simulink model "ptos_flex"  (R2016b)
settings: Solver=ode4  StartTime=0.0  StopTime=trun  FixedStep=step_sz  RelTol=1e-7  EnableMultiTasking=on
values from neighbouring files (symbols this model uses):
  A = [0 1;-(w)^2 0;]    [figure_4.m]    (also in figure_3.m; figure_2.m; results.m)
  alpha = .5    (= 0.5)    [figure_4.m]    (also in figure_3.m = 0.8; figure_2.m; results.m = 0.7)
  B = [0; bo]    [figure_4.m]    (also in figure_3.m; figure_2.m; results.m)
  bo = 1.8276*10^7    (= 18276000)    [figure_4.m]    (also in figure_3.m; figure_2.m; results.m)
  c = bo/w^2    (= 4.59233914625)    [figure_4.m]    (also in figure_3.m; figure_2.m; results.m)
  k1 = (c-xl)/(c*xl)    (= 1.95978557188)    [figure_4.m]    (also in figure_3.m = 0.508092555672; figure_2.m; results.m = 0.819169630574; switching_curves_comp_func.m = (c-xl)/(c*xl))
  k2 = sqrt(2*c*alpha*xl-alpha*xl^2)/(alpha*w*c*xl)    [figure_4.m]    (also in figure_3.m; figure_2.m; results.m; switching_curves_comp_func.m)
  T = 1    [figure_4.m]    (also in figure_3.m; figure_2.m; results.m; switching_curves_comp_func.m)
  w = 2*pi*3.175*10^2    (= 1994.91133503)    [figure_4.m]    (also in figure_3.m; figure_2.m; results.m; plotshaded.m = varargout)
  x2_bound = 10*bo/w    (= 91613.0941716)    [figure_4.m]    (also in figure_3.m; figure_2.m = 18322.6188343; results.m = 18322.6188343)
  xl = .1*c    (= 0.459233914625)    [figure_4.m]    (also in figure_3.m = 1.37770174388; figure_2.m; results.m = 0.964391220713)
  Xo = [8.665 4229]    [figure_4.m]    (also in figure_3.m = [2*c, 0]; figure_2.m = [curves_optx1(k), curves_optx2(k)]; results.m = [3.0*c,0])
libraries: simulink x3

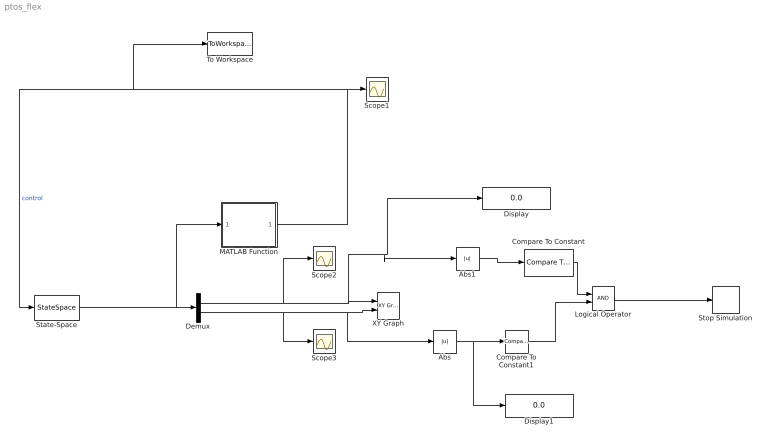
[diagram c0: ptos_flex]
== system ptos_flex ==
  Abs : Abs  Commented=on
  Abs1 : Abs  Commented=on
  Compare To Constant : simulink/Logic and Bit Operations/Compare To Constant  Commented=on  relop=<  const=2.6*10^-9  OutDataTypeStr=boolean
  Compare To Constant1 : simulink/Logic and Bit Operations/Compare To Constant  Commented=on  relop=<=  const=.1  OutDataTypeStr=boolean
  Demux : Demux  Outputs=[1, 1]
  Display : Display
  Display1 : Display
  Logical Operator : Logic  Commented=on  AllPortsSameDT=off  OutDataTypeStr=boolean
  MATLAB Function : MATLAB Function  TreatAsAtomicUnit=on
  Scope1 : Scope
  Scope2 : Scope
  Scope3 : Scope
  State-Space : StateSpace  A=A  B=B  C=eye(2)  D=[0;0]  X0=Xo  ContinuousStateAttributes="{'xx1',  'xx2'}"
  Stop Simulation : Stop  Commented=on
  To Workspace : ToWorkspace  VariableName=control_flex_ptos  SampleTime=-1
  XY Graph : simulink/Sinks/XY Graph  Commented=on  xmin=-25  xmax=25  ymin=-20000  ymax=20000  st=-1
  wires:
  Demux/1 -> Scope2/1, Abs1/1, Display/1, XY Graph/1
  Demux/2 -> Scope3/1, Abs/1, XY Graph/2
  State-Space/1 -> MATLAB Function/1(u), Demux/1
  MATLAB Function/1(y) -> Scope1/1, To Workspace/1, State-Space/1  "control"
  Compare To Constant/1 -> Logical Operator/1
  Logical Operator/1 -> Stop Simulation/1
  Compare To Constant1/1 -> Logical Operator/2
  Abs/1 -> Compare To Constant1/1, Display1/1
  Abs1/1 -> Compare To Constant/1

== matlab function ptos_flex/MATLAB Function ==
function y = fcn(u, bo, w, c, xl, k1, k2, T, alpha, x2_bound)
%#codegen



fArg=u(1)/c;
fpart=fArg-fix(fArg);

%% compute x1_bar
if (mod(sign(u(1)/c)*floor(abs(u(1)/c)), 2)==0);
        x1_bar=c-abs(fpart*c);
    else
        x1_bar=fpart*c;
    end

%% compute control
% <x2_bound
if( abs(u(1)) < 2*c & abs(u(1)) > xl )
      Fptos= sign(u(1)) *( w*sqrt(alpha*2*c*abs(u(1)) -alpha*u(1)^2) -1/k2);
      control=sat( k2*(-Fptos -u(2)), T);
 elseif(abs(u(1)) <xl )
     Fptos=(k1/k2)*u(1);
     control=sat( k2*(-Fptos -u(2)), T);

elseif( sign(u(1)*u(2))==1 | (u(2)/w)^2 <= (c^2 - x1_bar^2) )
    control=-sign(u(1));
else
    control=sign(u(1));
end



y=[control];
